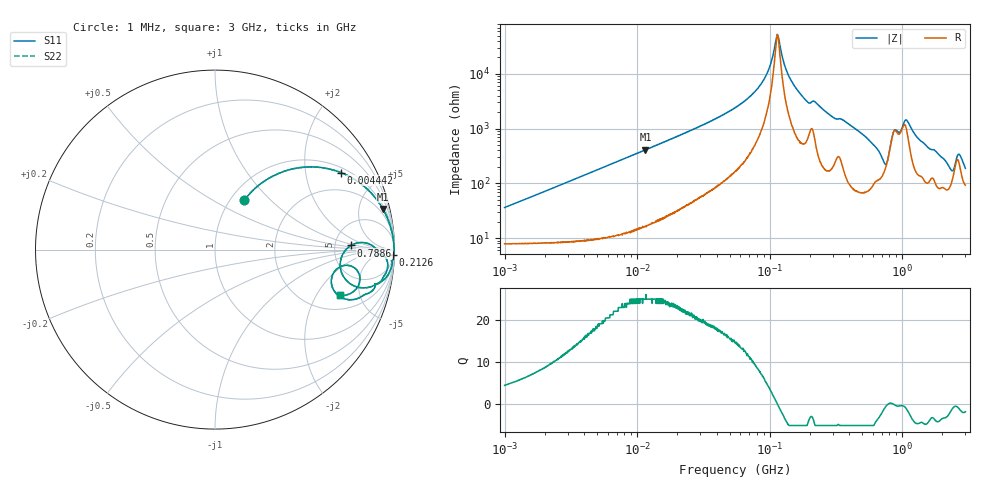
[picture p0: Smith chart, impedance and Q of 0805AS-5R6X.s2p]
!s-Parameter Generated by FASTRON Sdn. Bhd.
!FASTRON P/N : 0805AS-5R6X
!Keysight Technologies: E4991B_MY54100416_A.01.15
!Date: Mon Jun 15 12:59:42 2026
!Version  :Rev01  Mon Jun 15 12:59:42 2026
!Data & Calibration Information:
!Freq  S11  S21  S12  S22
!PortZ  Port1:50+j0  Port2:50+j0
!When reading reference impedance value at option line is always used.
! Remarks : This data is being provided solely for informational purposes.
# Hz S dB R 50
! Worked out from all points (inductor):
!   1601 points, 1 MHz to 3 GHz, reference 50 ohm
!   read as one part in series: L = 5.62 uH near 1.041 MHz
!   highest Q = 24.9 at 11.55 MHz (marker M1), where L = 5.65 uH
!   self-resonance near 114.3 MHz
!   S11 on the Smith chart (normalised r, x): 1 MHz: 1.16, +0.71; 4.442 MHz: 1.19, +3.13; 212.6 MHz: 19, -61; 788.6 MHz: 7.20, +0.78; 3 GHz: 2.86, -3.27
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1000000  -9.92 59.3  -1.10 -18.1  -1.10 -18.1  -9.92 59.3
3804036  -2.18 35.3  -4.75 -50.9  -4.75 -50.9  -2.18 35.3
4442361  -1.71 31.5  -5.62 -55.1  -5.62 -55.1  -1.71 31.5
1.155301e7  -0.33 13.6  -12.60 -74.1  -12.60 -74.1  -0.33 13.6
1.447069e7  -0.23 10.9  -14.50 -76.8  -14.50 -76.8  -0.23 10.9
5.504702e7  -0.03 2.4  -27.70 -83.7  -27.70 -83.7  -0.03 2.4
8.899408e7  -0.02 0.8  -37.40 -80.7  -37.40 -80.7  -0.02 0.8
9.984923e7  -0.02 0.4  -42.50 -74.6  -42.50 -74.6  -0.02 0.4
1.142934e8  -0.02 0.0  -54.40 -4.2  -54.40 -4.2  -0.02 0.0
1.43876e8  -0.02 -0.7  -38.00 79.4  -38.00 79.4  -0.02 -0.7
2.083556e8  -0.09 -1.7  -29.90 69.4  -29.90 69.4  -0.09 -1.7
2.125681e8  -0.08 -1.7  -30.10 71.9  -30.10 71.9  -0.08 -1.7
5.232078e8  -0.19 -7.7  -17.40 76.9  -17.40 76.9  -0.19 -7.7
6.924261e8  -1.26 -14.2  -11.50 52.9  -11.50 52.9  -1.26 -14.2
7.886361e8  -2.40 1.7  -12.30 -5.4  -12.30 -5.4  -2.40 1.7
7.925923e8  -2.27 2.2  -12.70 -7.2  -12.70 -7.2  -2.27 2.2
8.672962e8  -0.91 -0.2  -20.00 1.7  -20.00 1.7  -0.91 -0.2
1.070143e9  -0.43 -2.6  -23.60 40.9  -23.60 40.9  -0.43 -2.6
1.347129e9  -0.39 -8.5  -16.40 68.9  -16.40 68.9  -0.39 -8.5
2.278218e9  -2.31 -20.8  -8.11 43.9  -8.11 43.9  -2.31 -20.8
2.660507e9  -1.85 -9.0  -12.50 32.1  -12.50 32.1  -1.85 -9.0
3e9  -2.57 -20.1  -8.06 40.3  -8.06 40.3  -2.57 -20.1
